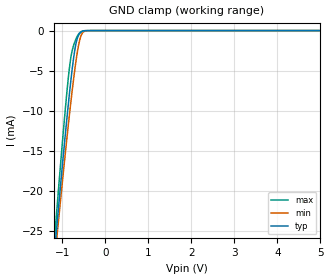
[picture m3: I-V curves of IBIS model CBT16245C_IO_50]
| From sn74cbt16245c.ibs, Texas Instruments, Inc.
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[Model]   CBT16245C_IO_50
Model_type  Terminator
| variable   typ   min   max
C_comp   6.31pF   4.26pF   12.73pF
| C_tri-state   6.31pF   4.26pF   12.73pF
[Temperature Range]   40   100   -40
| Ambient temperature   25   85   -40
[Voltage range]   5   4.5   5.5
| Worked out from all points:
|   GND clamp passes 1 mA (typ) near -0.65 V on its own axis
[GND Clamp]
| CBT16245C_IO_50
|   Voltage   I(typ)   I(min)   I(max)
-5V       -286.9mA   -267.5mA   -309.2mA
-1.19V    -28.47mA   -29.59mA   -26.88mA
-1.155V   -26.34mA   -27.64mA   -24.51mA
-1.12V    -24.23mA   -25.7mA    -22.17mA
-1.085V   -22.14mA   -23.78mA   -19.85mA
-925mV    -12.91mA   -15.26mA   -9.733mA
-815mV    -7.1mA     -9.758mA   -4.012mA
-760mV    -4.528mA   -7.197mA   -2.356mA
-675mV    -1.54mA    -3.676mA   -1.013mA
-610mV    -508.2uA   -1.614mA   -383.4uA
-545mV    -149.1uA   -450.9uA   -90.44uA
5V        473.9pA    1.464nA    157.4pA
